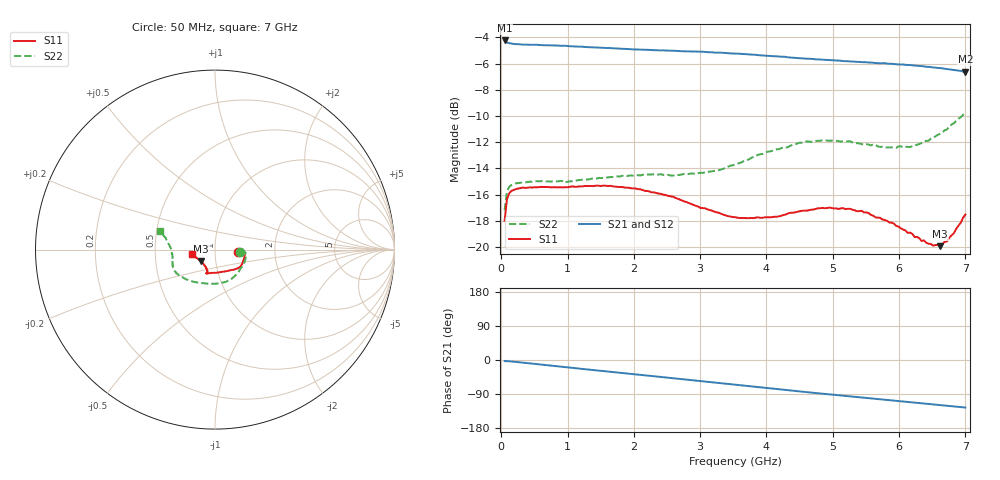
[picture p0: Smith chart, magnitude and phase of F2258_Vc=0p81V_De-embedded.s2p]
! Integrated Device Technology
! Corporate Headquarters
! 6024 Silver Creek Valley Road
! San Jose, CA 95138  USA
! Phone:  1-408-284-8200
! Toll Free:  1-800-223-1366
! Webpage:  http://www.idt.com/
! Timing and RF Division
! 515 Groton Road, Suite 102
! Westford, MA 01886-6024
! Device:  F2258
! Description: Voltage Variable RF Attenuator
! Frequency:  50.0 -  6000.00 MHz
! Package:  3x3 mm Thin QFN Plastic Package: 16 pin
! Ports:  2 RF, 2 DC
!  Pin  1  = NC
!  Pin  2  = NC
!  Pin  3  = RF2  = Port 2
!  Pin  4  = GND
!  Pin  5  = Vdd
!  Pin  6  = NC
!  Pin  7  = VCTRL
!  Pin  8  = NC
!  Pin  9  = GND
!  Pin 10  = RF1  = Port 1
!  Pin 11  = NC
!  Pin 12  = NC
!  Pin 13  = NC
!  Pin 14  = NC
!  Pin 15  = NC
!  Pin 16  = NC
! Vcntrl:  0.810 Volts
! Vdd:  +3.300 Volts
! Current:  1.134 mA
! Data:  The device was measured on a the F2258 evaluation board which has
!  individual transmission lines to the RF pins.  Data was collected
!  using a calibrated network analyzer.  The evaluation board was
!  de-embedded using a TRL calibration technique.
!  The reference plane is the edge of the package pin.
! Misc:  SN 10
!  Action Tracker AT0285
! Date Measured:  2014-12-10
! Date:  2016-01-13  MJV
! Note:
!  Integrated Device Technology supplies this data as a sample of measured
!  data at the package pin for this product.  Your particular data for this
!  product may vary.
!  Data was taken at 25 degrees C.
!  Integrated Device Technology reserves the right to change this data at anytime.
!Freq_(GHz)  S11M_(dB)  S11P_(deg)  S21M_(dB)  S21P_(deg)  S12M_(dB)  S12P_(deg)  S22M_(dB)  S22P_(deg)
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# GHz S dB R 50
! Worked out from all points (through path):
!   201 points, 50 MHz to 7 GHz, reference 50 ohm
!   highest |S21| = -4.23 dB at 50 MHz (marker M1); lowest = -6.6 dB at 7 GHz (marker M2)
!   group delay of S21, straight-line fit = 49.6 ps
!   lowest |S11| = -19.9 dB at 6.618 GHz (marker M3), VSWR 1.22, Z = 42.5 - j5.5 ohm
!   |S11| at or under -10 dB: start of sweep to end of sweep
!   |S22| runs from -17.2 to -9.7 dB; largest |S21 - S12| = 0.0026
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0.05  -18.00 -5.0  -4.23 -2.9  -4.22 -2.9  -17.21 -5.3
0.08475  -16.37 -3.6  -4.38 -3.0  -4.36 -3.0  -15.78 -4.6
0.1195  -15.90 -3.5  -4.44 -3.4  -4.41 -3.4  -15.41 -5.3
0.15425  -15.71 -4.0  -4.47 -3.9  -4.45 -3.9  -15.27 -6.5
0.606  -15.41 -13.7  -4.59 -12.2  -4.59 -12.2  -14.97 -21.7
0.9535  -15.44 -22.1  -4.64 -18.6  -4.64 -18.6  -15.09 -34.3
1.2315  -15.38 -26.8  -4.71 -23.7  -4.72 -23.7  -14.85 -43.3
1.6485  -15.33 -32.9  -4.81 -31.2  -4.82 -31.2  -14.66 -55.3
2.37825  -15.92 -41.8  -4.99 -44.2  -4.99 -44.2  -14.46 -75.1
2.93425  -16.85 -52.9  -5.09 -54.4  -5.08 -54.4  -14.42 -93.5
3.525  -17.73 -73.4  -5.23 -65.3  -5.24 -65.3  -13.71 -116.7
4.11575  -17.70 -96.3  -5.44 -76.2  -5.44 -76.1  -12.59 -137.1
4.498  -17.28 -105.9  -5.59 -83.0  -5.57 -83.0  -12.04 -146.8
4.7065  -17.14 -108.1  -5.65 -86.6  -5.65 -86.6  -11.96 -150.9
4.94975  -16.99 -109.6  -5.73 -90.7  -5.73 -90.7  -11.88 -155.0
5.43625  -17.23 -109.5  -5.89 -98.9  -5.88 -98.9  -12.15 -162.9
5.85325  -18.13 -110.3  -6.02 -105.9  -6.01 -106.0  -12.39 -171.3
6.166  -18.90 -115.5  -6.11 -111.3  -6.11 -111.3  -12.38 -178.5
6.33975  -19.55 -121.9  -6.19 -114.4  -6.23 -114.4  -12.07 176.8
6.61775  -19.94 -140.5  -6.34 -119.1  -6.37 -119.1  -11.36 169.5
6.82625  -18.96 -156.1  -6.49 -122.7  -6.50 -122.6  -10.56 164.7
7  -17.53 -168.7  -6.63 -125.5  -6.66 -125.5  -9.73 161.0
